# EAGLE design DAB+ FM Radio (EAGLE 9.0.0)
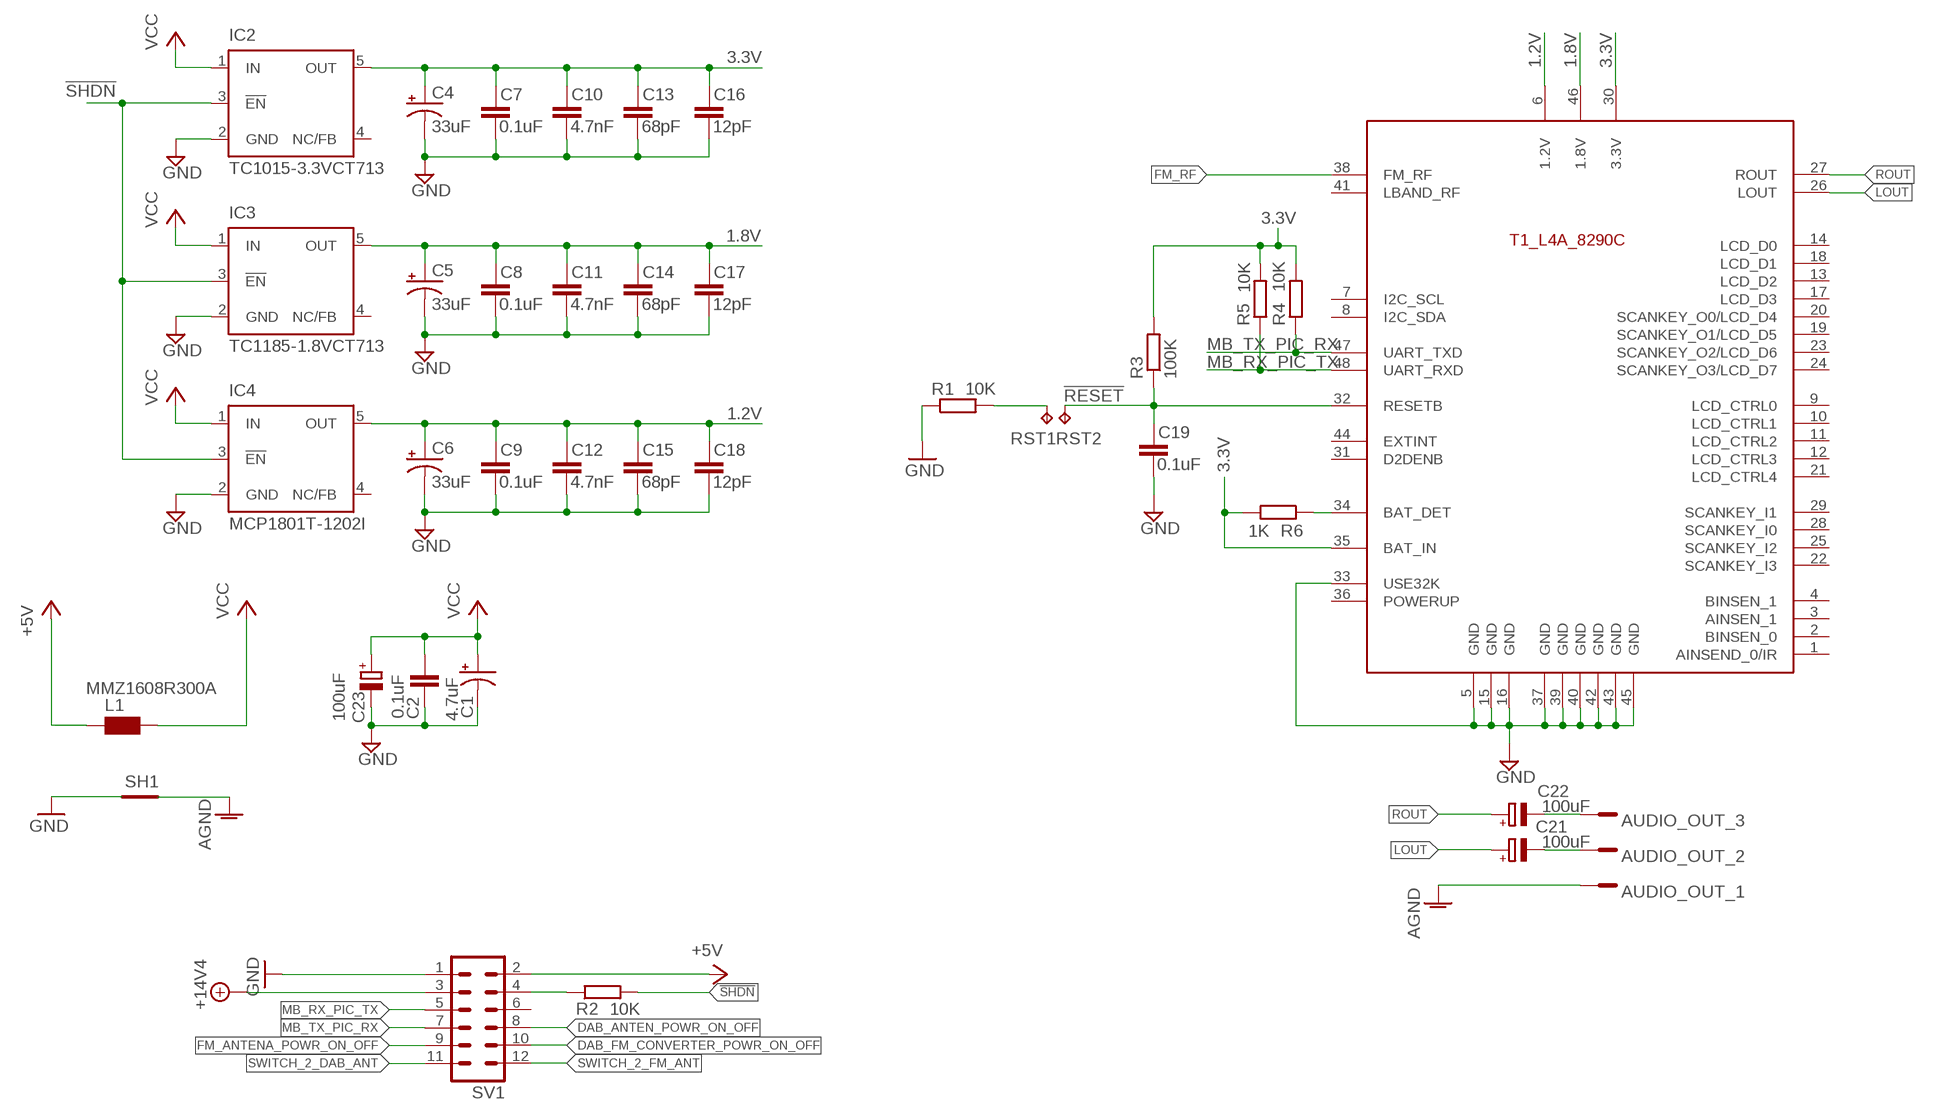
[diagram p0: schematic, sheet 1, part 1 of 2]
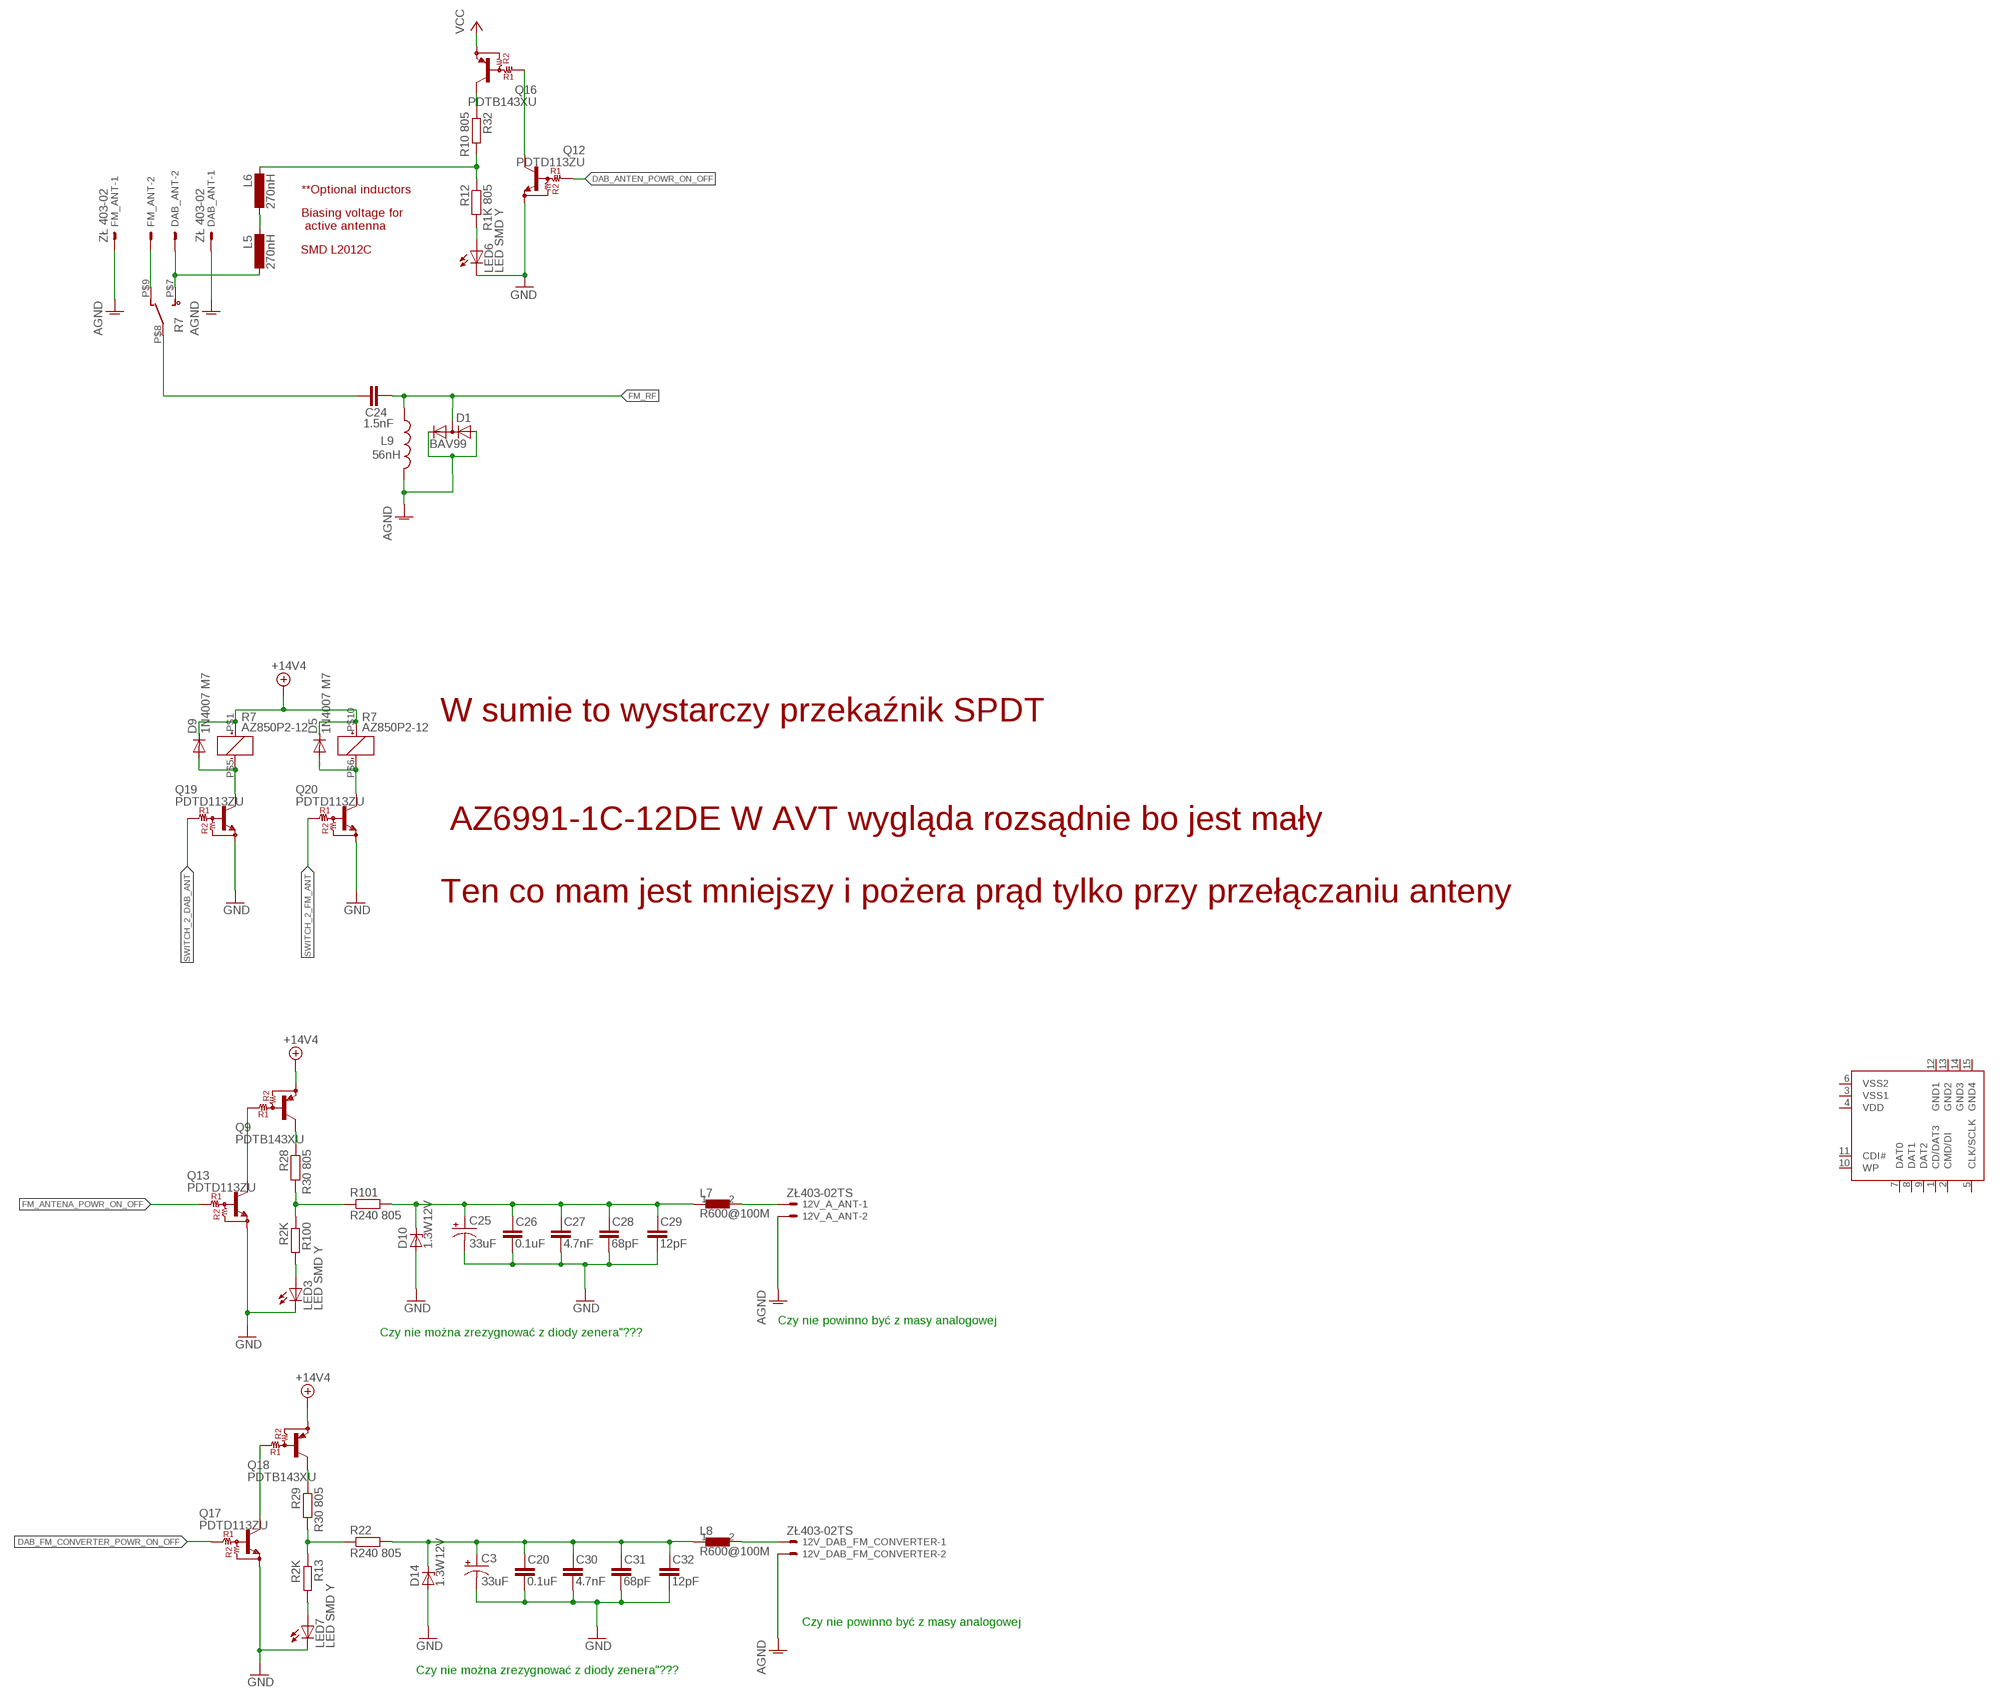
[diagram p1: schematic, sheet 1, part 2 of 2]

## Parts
12V_A_ANT  ZŁ403-02TS  22-23-2021  [22-23-2021]
12V_DAB_FM_CONVERTER  ZŁ403-02TS  22-23-2021  [22-23-2021]
AUDIO_OUT  JST_3_PIN_B3B-PH-KS  [B3B-PH-KS]
C1  4.7uF  CAP_POL1206  [EIA3216]
C2  0.1uF  C-EUC0603  [C0603]
C3  33uF  CAP_POL1206  [EIA3216]
C4  33uF  CAP_POL1206  [EIA3216]
C5  33uF  CAP_POL1206  [EIA3216]
C6  33uF  CAP_POL1206  [EIA3216]
C7  0.1uF  C-EUC0603  [C0603]
C8  0.1uF  C-EUC0603  [C0603]
C9  0.1uF  C-EUC0603  [C0603]
C10  4.7nF  C-EUC0603  [C0603]
C11  4.7nF  C-EUC0603  [C0603]
C12  4.7nF  C-EUC0603  [C0603]
C13  68pF  C-EUC0603  [C0603]
C14  68pF  C-EUC0603  [C0603]
C15  68pF  C-EUC0603  [C0603]
C16  12pF  C-EUC0603  [C0603]
C17  12pF  C-EUC0603  [C0603]
C18  12pF  C-EUC0603  [C0603]
C19  0.1uF  C-EUC0603  [C0603]
C20  0.1uF  C-EUC0603  [C0603]
C21  100uF  CPOL-EUD  [PANASONIC_D]
C22  100uF  CPOL-EUD  [PANASONIC_D]
C23  100uF  CPOL-EUD  [PANASONIC_D]
C24  1.5nF  C-EUC0603  [C0603]
C25  33uF  CAP_POL1206  [EIA3216]
C26  0.1uF  C-EUC0603  [C0603]
C27  4.7nF  C-EUC0603  [C0603]
C28  68pF  C-EUC0603  [C0603]
C29  12pF  C-EUC0603  [C0603]
C30  4.7nF  C-EUC0603  [C0603]
C31  68pF  C-EUC0603  [C0603]
C32  12pF  C-EUC0603  [C0603]
D1  BAV99  BAV199  [SOT23]
D5  1N4007 M7  CGRM4001-G  [SOD-123_MINI-SMA]
D9  1N4007 M7  CGRM4001-G  [SOD-123_MINI-SMA]
D10  1.3W12V  ZENER-DIODEZD-2.5  [ZDIO-2.5]
D14  1.3W12V  ZENER-DIODEZD-2.5  [ZDIO-2.5]
DAB_ANT  ZŁ 403-02  22-27-2021-02  [6410-02]
FM_ANT  ZŁ 403-02  22-27-2021-02  [6410-02]
IC2  TC1015-3.3VCT713  TPS77001  [SOT23-DBV]
IC3  TC1185-1.8VCT713  TPS77001  [SOT23-DBV]
IC4  MCP1801T-1202I  TPS77001  [SOT23-DBV]
L1  MMZ1608R300A  WE-CBF_0603  [0603]
L5  270nH  L-EUL2012C  [L2012C]
L6  270nH  L-EUL2012C  [L2012C]
L7  R600@100M  FERRITR0805  [R0805]
L8  R600@100M  FERRITR0805  [R0805]
L9  56nH  INDUCTOR0603  [0603]
LED3  LED SMD Y  LED  [SMARTLED-TTW]
LED6  LED SMD Y  LED  [SMARTLED-TTW]
LED7  LED SMD Y  LED  [SMARTLED-TTW]
Q9  PDTB143XU  [SOT-23]
Q12  PDTD113ZU  [SOT-23]
Q13  PDTD113ZU  [SOT-23]
Q16  PDTB143XU  [SOT-23]
Q17  PDTD113ZU  [SOT-23]
Q18  PDTB143XU  [SOT-23]
Q19  PDTD113ZU  [SOT-23]
Q20  PDTD113ZU  [SOT-23]
R1  10K  R-EU_R0603  [R0603]
R2  10K  R-EU_R0603  [R0603]
R3  100K  R-EU_R0603  [R0603]
R4  10K  R-EU_R0603  [R0603]
R5  10K  R-EU_R0603  [R0603]
R6  1K  R-EU_R0603  [R0603]
R7  AZ850P2-12  [AZ850-2C]
R12  R1K 805  R-EU_R0805  [R0805]
R13  R2K  R-EU_R0805  [R0805]
R22  R240 805  R-EU_M0805  [M0805]
R28  R30 805  R-EU_R0805  [R0805]
R29  R30 805  R-EU_R0805  [R0805]
R32  R10 805  R-EU_R0805  [R0805]
R100  R2K  R-EU_R0805  [R0805]
R101  R240 805  R-EU_M0805  [M0805]
RST1  TPB1,27  [B1,27]
RST2  TPB1,27  [B1,27]
SH1  SHORT-HT5  [SHORT_TOP-50]
SV1  MA06-2  [MA06-2]
U$1  T1_L4A_8290C/T2_L4A_8650C  T1_L4A_8290C  [T1_L4A]
U$6  ZŁ KART SD  SDCARDVAR2  [SDCMF-10915W010]

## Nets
1.2V: C6.A(+) C9.1 C12.1 C15.1 C18.1 IC4.5(OUT) U$1.6(1.2V)
1.8V: C5.A(+) C8.1 C11.1 C14.1 C17.1 IC3.5(OUT) U$1.46(1.8V)
3.3V: C4.A(+) C7.1 C10.1 C13.1 C16.1 IC2.5(OUT) R3.2 R4.2 R5.2 R6.2 U$1.30(3.3V) U$1.35(BAT_IN)
!RESET!: C19.1 R3.1 RST2.TP U$1.32(RESETB)
!SHDN!: IC2.3(!EN) IC3.3(!EN) IC4.3(!EN) R2.2
+5V: L1.1 SV1.2
+12V: D5.C D9.C Q9.2(E) Q18.2(E) R7.P$1(S$1:+) R7.P$10(R$2:+) SV1.3 ; supply symbol labelled +14V4
AGND: 12V_A_ANT.2 12V_DAB_FM_CONVERTER.2 AUDIO_OUT.P$1 D1.1(A) D1.2(C) DAB_ANT.1 FM_ANT.1 L9.2 SH1.2
DAB_ANTEN_POWR_ON_OFF: Q12.1(B) SV1.8
DAB_FM_CONVERTER_POWR_ON_OFF: Q17.1(B) SV1.10
FM_ANTENA_POWR_ON_OFF: Q13.1(B) SV1.9
FM_RF: C24.2 D1.3(AC) L9.1 U$1.38(FM_RF)
GND: C1.C(-) C2.2 C3.C(-) C4.C(-) C5.C(-) C6.C(-) C7.2 C8.2 C9.2 C10.2 C11.2 C12.2 C13.2 C14.2 C15.2 C16.2 C17.2 C18.2 C19.2 C20.2 C23.- C25.C(-) C26.2 C27.2 C28.2 C29.2 C30.2 C31.2 C32.2 D10.A D14.A IC2.2(GND) IC3.2(GND) IC4.2(GND) LED3.C@1(C) LED6.C@1(C) LED7.C@1(C) Q12.2(E) Q13.2(E) Q17.2(E) Q19.2(E) Q20.2(E) R1.1 SH1.1 SV1.1 U$1.5(GND) U$1.15(GND) U$1.16(GND) U$1.33(USE32K) U$1.37(GND) U$1.39(GND) U$1.40(GND) U$1.42(GND) U$1.43(GND) U$1.45(GND)
LOUT: C21.+ U$1.26(LOUT)
MB_RX_PIC_TX: R5.1 SV1.5 U$1.48(UART_RXD)
MB_TX_PIC_RX: R4.1 SV1.7 U$1.47(UART_TXD)
N$1: D5.A Q20.3(C) R7.P$6(R$2:-)
N$2: D9.A Q19.3(C) R7.P$5(S$1:-)
N$3: R6.1 U$1.34(BAT_DET)
N$4: C24.1 R7.P$8
N$5: DAB_ANT.2 L5.2 R7.P$7
N$6: AUDIO_OUT.P$3 C22.-
N$7: FM_ANT.2 R7.P$9
N$8: AUDIO_OUT.P$2 C21.-
N$9: L6.1 R12.1 R32.2
N$10: R2.1 SV1.4
N$12: L5.1 L6.2
N$13: R1.2 RST1.TP
N$20: Q12.3(C) Q16.1(B)
N$23: LED6.A@1(A) R12.2
N$25: Q17.3(C) Q18.1(B)
N$26: R13.1 R22.1 R29.2
N$27: LED7.A@1(A) R13.2
N$29: C3.A(+) C20.1 C30.1 C31.1 C32.1 D14.C L8.1 R22.2
N$30: 12V_DAB_FM_CONVERTER.1 L8.2
N$33: Q16.3(C) R32.1
N$34: Q9.3(C) R28.1
N$35: Q18.3(C) R29.1
N$85: Q9.1(B) Q13.3(C)
N$87: R28.2 R100.1 R101.1
N$88: LED3.A@1(A) R100.2
N$91: C25.A(+) C26.1 C27.1 C28.1 C29.1 D10.C L7.1 R101.2
N$92: 12V_A_ANT.1 L7.2
ROUT: C22.+ U$1.27(ROUT)
SWITCH_2_DAB_ANT: Q19.1(B) SV1.11
SWITCH_2_FM_ANT: Q20.1(B) SV1.12
VCC: C1.A(+) C2.1 C23.+ IC2.1(IN) IC3.1(IN) IC4.1(IN) L1.2 Q16.2(E)
Unconnected: IC2.4(NC/FB) IC3.4(NC/FB) IC4.4(NC/FB) R7.P$2 R7.P$3 R7.P$4 SV1.6 U$1.1(AINSEND_0/IR) U$1.2(BINSEN_0) U$1.3(AINSEN_1) U$1.4(BINSEN_1) U$1.7(I2C_SCL) U$1.8(I2C_SDA) U$1.9(LCD_CTRL0) U$1.10(LCD_CTRL1) U$1.11(LCD_CTRL2) U$1.12(LCD_CTRL3) U$1.13(LCD_D2) U$1.14(LCD_D0) U$1.17(LCD_D3) U$1.18(LCD_D1) U$1.19(SCANKEY_O1/LCD_D5) U$1.20(SCANKEY_O0/LCD_D4) U$1.21(LCD_CTRL4) U$1.22(SCANKEY_I3) U$1.23(SCANKEY_O2/LCD_D6) U$1.24(SCANKEY_O3/LCD_D7) U$1.25(SCANKEY_I2) U$1.28(SCANKEY_I0) U$1.29(SCANKEY_I1) U$1.31(D2DENB) U$1.36(POWERUP) U$1.41(LBAND_RF) U$1.44(EXTINT) U$6.1(CD/DAT3) U$6.2(CMD/DI) U$6.5(CLK/SCLK) U$6.7(DAT0) U$6.8(DAT1) U$6.9(DAT2) U$6.10(WP) U$6.11(CDI#)

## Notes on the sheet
- **Optional inductors
- Biasing voltage for
   active antenna
- SMD L2012C
- W sumie to wystarczy przekaźnik SPDT
  
  
   AZ6991-1C-12DE W AVT wygląda rozsądnie bo jest mały
  
  Ten co mam jest mniejszy i pożera prąd tylko przy przełączaniu anteny
- Czy nie powinno być z masy analogowej
- Czy nie można zrezygnować z diody zenera"???
- Czy nie powinno być z masy analogowej
- Czy nie można zrezygnować z diody zenera"???

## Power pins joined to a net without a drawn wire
GND1: U$6.12(GND1)
GND2: U$6.13(GND2)
GND3: U$6.14(GND3)
GND4: U$6.15(GND4)
VDD: U$6.4(VDD)
VSS1: U$6.3(VSS1)
VSS2: U$6.6(VSS2)

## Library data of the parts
12V_A_ANT 12V_DAB_FM_CONVERTER = con-molex:22-23-2021: .100" (2.54mm) Center Header - 2 Pin; MF: MOLEX; MPN: 22-23-2021; OC_FARNELL: 1462926; OC_NEWARK: 25C3832
AUDIO_OUT = conn-JST:JST_3_PIN_
C1 C3-C6 C25 = SparkFun:CAP_POL: Capacitor Polarized
C2 C7-C20 C24 C26-C32 = rcl:C-EU: CAPACITOR, European symbol
C21-C23 = rcl:CPOL-EU: POLARIZED CAPACITOR, European symbol
D1 = diode:BAV199: DIODE low-leakage double diode
D5 D9 = diode:CGRM400*-G: Molded plasitc,JEDEC SOD-123/Mini SMA
D10 D14 = diode:ZENER-DIODE: Z-Diode
DAB_ANT FM_ANT = con-molex:22-?-02: CONNECTOR; OC_FARNELL: unknown; OC_NEWARK: unknown
IC2-IC4 = texas:TPS770*: ULTRALOW-POWER 50-mA LOW-DROPOUT LINEAR REGULATORS 50-mA Low-Dropout Regulator Source: http://focus.ti.com/lit/ds/symlink/tps77001.pdf; MF: TEXAS INSTRUMENTS; MPN: TPS77001DBVT; OC_FARNELL: 8461554; OC_NEWARK: 77C1171
L1 = wuerth-elektronik:WE-CBF: SMD EMI Suppression Ferrite Beads
L5 L6 = resistor:L-EU: INDUCTOR, European symbol
L7 L8 = ferrit_bear:FERRIT
L9 = SparkFun:INDUCTOR: Inductors
LED3 LED6 LED7 = adafruit:LED: LED
Q9 Q16 Q18 = pre-bias-transistor:PDTB: PNP Resistor-Equipped Transistor (RET) family in a very small SOT323 (SC-70) Surface-Mounted Device (SMD) plastic package. VCC = -50 IC (max) = -500mA; R1: 4.7 kOhm; R2: 10 kOhm
Q12 Q13 Q17 Q19 Q20 = pre-bias-transistor:PDTD: Pre biase NPN transistor NPN Resistor-Equipped Transistor (RET) family in a very small SOT323 (SC-70) Surface-Mounted Device (SMD) plastic package. VCC = 50V Ic (max) = 500 mA; R1: 1 kOhm; R2: 10 kOhm
R1-R6 R12 R13 R22 R28 R29 R32 R100 R101 = rcl:R-EU_: RESISTOR, European symbol
R7 = relay_silelis:AZ850P2-12
RST1 RST2 = testpad:TP: Test pad
SH1 = shorts-old:SHORT-H: Short between two nets; BOM: no
SV1 = con-lstb:MA06-2: PIN HEADER; OC_FARNELL: unknown; OC_NEWARK: unknown
U$1 = Monkey:T1_L4A_8290C
U$6 = kingfont_sdcmf10915w010_covek:SDCARD: SD card connector KINGFONT SDCMF-10915W010

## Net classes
0 default: clearance 0.203 mm

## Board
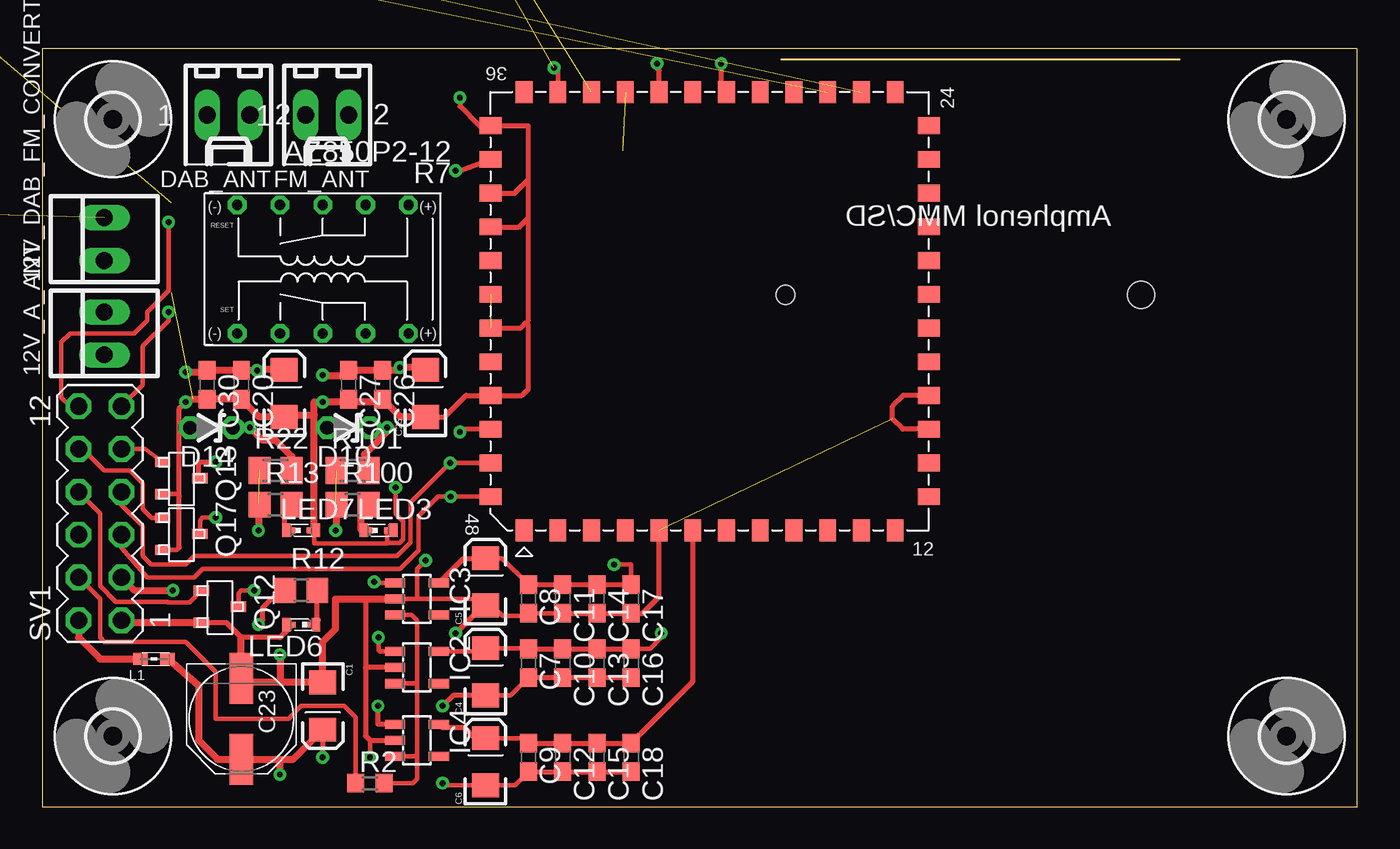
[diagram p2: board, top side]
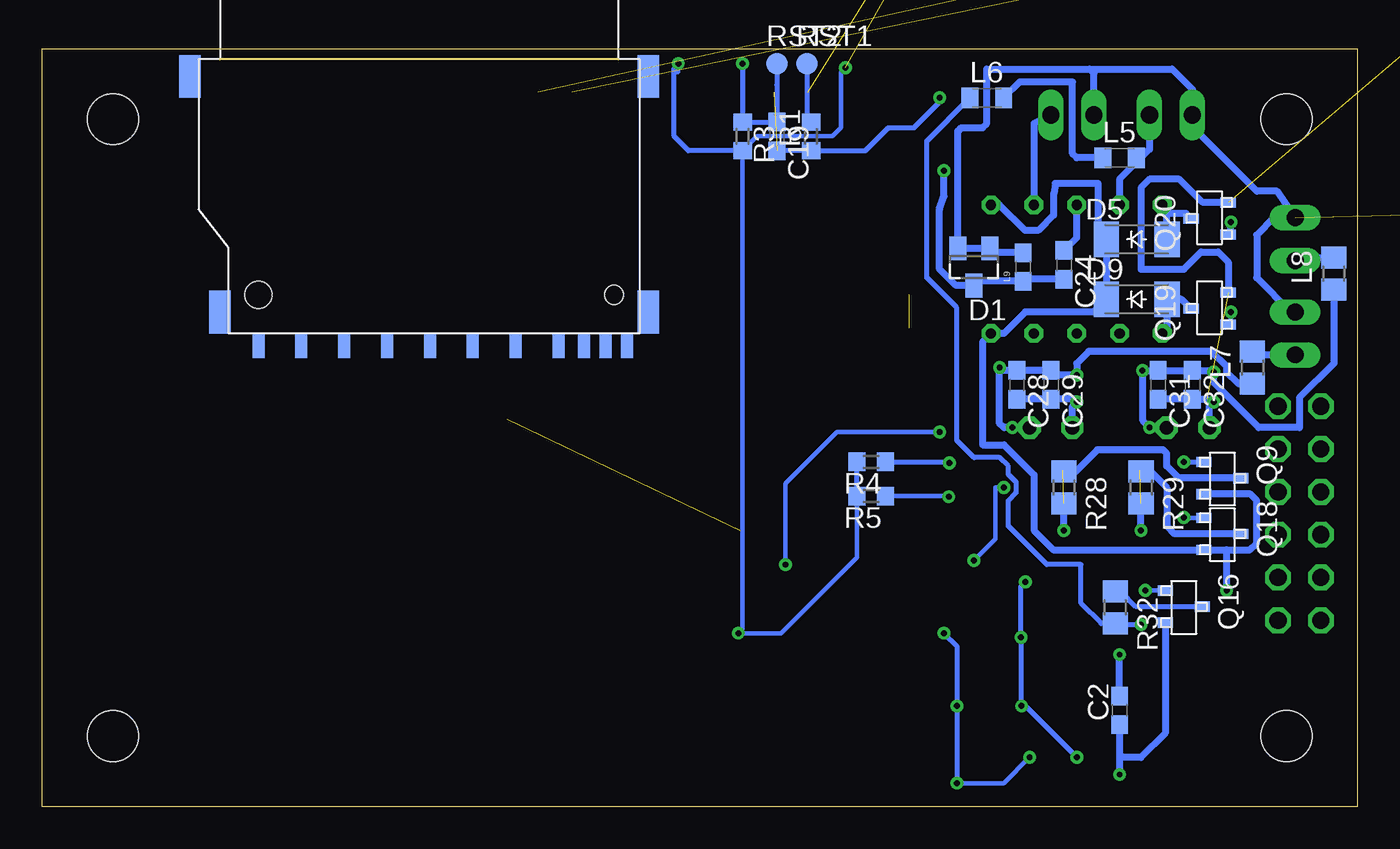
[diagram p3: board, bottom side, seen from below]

Size 77.98 x 44.96 mm. Coordinates in mm from the lower left corner, seen from the top.
Outline: 0,0 77.98,0 77.98,44.96 0,44.96 0,0
Copper layers (1*16): Top 0.035mm / dielectric 1.5mm / Bottom 0.035mm
Design rules "default": minimum track width 6mil, minimum drill 0.35mm, track to track 6mil, track to pad 6mil, pad to pad 6mil, via to via 6mil, smd to smd 6mil, copper to edge 40mil, drill to drill 6mil, minimum pad ring 10mil, minimum via ring 8mil, stop-mask expansion 4mil, vias tented up to drill 0mil, thermal gap 10mil

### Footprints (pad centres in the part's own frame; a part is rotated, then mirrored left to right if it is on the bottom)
22-23-2021 = drill 1 long: 1 -1.27,0; 2 1.27,0
B3B-PH-KS = drill 0.75 pad 1.2 square: P$1 -2,1.7; P$2 -4,1.7; P$3 -6,1.7
EIA3216 = smd 1.4 x 1.6: A 1.4,0; C -1.4,0
C0603 = smd 1.1 x 1: 1 -0.85,0; 2 0.85,0
PANASONIC_D = smd 3 x 1.4: + 2.4,0; - -2.4,0
SOT23 = smd 1 x 1.4: 1 -0.95,-1.1; 2 0.95,-1.1; 3 0,1.1
SOD-123_MINI-SMA = smd 1.5 x 2.1: A 1.8,0; C -1.8,0
ZDIO-2.5 = drill 0.813 octagon: A 1.27,0; C -1.27,0
6410-02 = drill 1.016 long: 1 1.27,0; 2 -1.27,0
SOT23-DBV = smd 0.55 x 1.2: 1 -0.95,-1.3; 2 0,-1.3; 3 0.95,-1.3; 4 0.95,1.3; 5 -0.95,1.3
0603 = smd 0.85 x 0.7: 1 -0.9,0; 2 0.7,0
L2012C = smd 1 x 1.2: 1 -1,0; 2 1,0
R0805 = smd 1.3 x 1.5: 1 -0.95,0; 2 0.95,0
0603' = smd 1.1 x 1: 1 -0.85,0; 2 0.85,0
SMARTLED-TTW = smd 0.8 x 0.5: A 0,-0.875; C 0,0.875 | smd 0.35 x 0.35: A@1 0,-0.5; C@1 0,0.5
SOT-23 = smd 0.6 x 0.9: 1 -1,-1.1; 2 0.9,-1.1; 3 -0.05,1.1
R0603 = smd 1 x 1.1: 1 -0.85,0; 2 0.85,0
AZ850-2C = drill 0.6 octagon: P$1 -5.08,3.81; P$2 -2.54,3.81; P$3 0,3.81; P$4 2.54,3.81; P$5 5.08,3.81; P$6 5.08,-3.81; P$7 2.54,-3.81; P$8 0,-3.81; P$9 -2.54,-3.81; P$10 -5.08,-3.81
M0805 = smd 1.3 x 1.6: 1 -0.95,0; 2 0.95,0
B1,27 = smd 1.27 x 1.27: TP 0,0
SHORT_TOP-50 = smd 1.27 x 1.27: 1 0.635,0; 2 -0.635,0
MA06-2 = drill 1.016 octagon: 1 -6.35,-1.27; 2 -6.35,1.27; 3 -3.81,-1.27; 4 -3.81,1.27; 5 -1.27,-1.27; 6 -1.27,1.27; 7 1.27,-1.27; 8 1.27,1.27; 9 3.81,-1.27; 10 3.81,1.27; 11 6.35,-1.27; 12 6.35,1.27
T1_L4A = smd 1.3 x 1: 1 0,0; 2 0,-2; 3 0,-4; 4 0,-6; 5 0,-8; 6 0,-10; 7 0,-12; 8 0,-14; 9 0,-16; 10 0,-18; 11 0,-20; 12 0,-22; 25 26,-22; 26 26,-20; 27 26,-18; 28 26,-16; 29 26,-14; 30 26,-12; 31 26,-10; 32 26,-8; 33 26,-6; 34 26,-4; 35 26,-2; 36 26,0 | smd 1 x 1.3: 13 2,-24; 14 4,-24; 15 6,-24; 16 8,-24; 17 10,-24; 18 12,-24; 19 14,-24; 20 16,-24; 21 18,-24; 22 20,-24; 23 22,-24; 24 24,-24; 37 24,2; 38 22,2; 39 20,2; 40 18,2; 41 16,2; 42 14,2; 43 12,2; 44 10,2; 45 8,2; 46 6,2; 47 4,2; 48 2,2
3,0 = hole 3: 0,0
SDCMF-10915W010 = smd 0.711 x 1.422: 1 7.366,13.462; 2 4.826,13.462; 3 2.286,13.462; 4 -0.254,13.462; 5 -2.794,13.462; 6 -5.334,13.462; 7 -7.874,13.462; 8 -9.398,13.462; 9 9.906,13.462; 10 -11.938,13.462; 11 -10.668,13.462 | smd 1.27 x 2.54: 12 12.192,11.43; 13 13.97,-2.54; 14 -13.208,-2.54; 15 -13.208,11.43 | hole 1.6: 9.906,10.414 | hole 1.1: -11.176,10.414

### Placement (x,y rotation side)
12V_A_ANT  3.68,28.07 90 top
12V_DAB_FM_CONVERTER  3.68,33.66 90 top
AUDIO_OUT  not placed on the board
C1  16.64,5.97 270 top
C2  14.1,5.71 90 bottom
C3  14.35,24.51 90 top
C4  26.29,8 90 top
C5  26.29,13.34 90 top
C6  26.29,2.67 90 top
C7  28.83,8.51 270 top
C8  28.83,12.32 270 top
C9  28.83,2.92 270 top
C10  30.86,8.51 270 top
C11  30.86,12.32 270 top
C12  30.86,2.92 270 top
C13  32.89,8.51 270 top
C14  32.89,12.32 270 top
C15  32.89,2.92 270 top
C16  34.92,8.51 270 top
C17  34.92,12.32 270 top
C18  34.92,2.92 270 top
C19  34.42,39.75 270 bottom
C20  11.81,25.02 270 top
C21  not placed on the board
C22  not placed on the board
C23  11.81,5.21 270 top
C24  17.4,32.13 270 bottom
C25  22.73,24.51 90 top
C26  20.19,25.02 270 top
C27  18.16,25.02 270 top
C28  20.19,25.02 270 bottom
C29  18.16,25.02 270 bottom
C30  9.78,25.02 270 top
C31  11.81,25.02 270 bottom
C32  9.78,25.02 270 bottom
D1  22.73,32 180 bottom
D5  13.08,33.66 0 bottom
D9  13.08,30.1 0 bottom
D10  18.16,22.48 180 top
D14  10.03,22.48 180 top
DAB_ANT  11.05,41.02 180 top
FM_ANT  16.89,41.02 180 top
IC2  22.22,8.25 270 top
IC3  22.22,12.32 270 top
IC4  22.22,3.94 270 top
L1  6.73,8.76 0 top
L5  14.1,38.48 0 bottom
L6  21.97,42.04 0 bottom
L7  6.22,26.04 90 bottom
L8  1.4,31.62 90 bottom
L9  56nH  [0603']  19.81,32 90 bottom
LED3  19.94,16.38 270 top
LED6  15.37,10.79 90 top
LED7  15.37,16.38 270 top
Q9  8,19.43 270 bottom
Q12  10.54,11.81 270 top
Q13  8.25,19.43 270 top
Q16  10.29,11.81 270 bottom
Q17  8.25,16.13 270 top
Q18  8,16.13 270 bottom
Q19  8.76,29.59 90 bottom
Q20  8.76,34.92 90 bottom
R1  32.38,39.75 90 bottom
R2  19.43,1.4 0 top
R3  36.45,39.75 270 bottom
R4  28.83,20.45 180 bottom
R5  28.83,18.41 180 bottom
R6  not placed on the board
R7  16.64,31.88 180 top
R12  15.37,12.83 0 top
R13  13.84,17.91 0 top
R22  13.84,19.94 0 top
R28  17.4,18.92 270 bottom
R29  12.83,18.92 270 bottom
R32  14.35,11.81 270 bottom
R100  18.41,17.91 0 top
R101  18.41,19.94 0 top
RST1  32.64,44.07 0 bottom
RST2  34.42,44.07 0 bottom
SH1  not placed on the board
SV1  3.43,17.4 90 top
U$1  28.57,16.38 90 top
U$2  [3,0]  4.19,40.77 0 top
U$3  [3,0]  4.19,4.19 0 top
U$4  [3,0]  73.79,40.77 0 top
U$5  [3,0]  73.79,4.19 0 top
U$6  55.24,40.77 180 bottom

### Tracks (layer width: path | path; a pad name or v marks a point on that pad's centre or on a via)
1.2V
  Top 0.254: C6.A 28.53,4.07 C9.1
  Top 0.305: IC4.5 23.71,4.7 25.02,4.7 25.65,4.07 C6.A 26.58,3.77 | C9.1 C12.1 C15.1 C18.1 38.57,7.42 U$1.6
1.8V  (via drill 0.35)
  Top 0.254: C5.A 27.26,14.73 C8.1 | C17.1 34.92,14.35 v33.91,14.35 | v24.77,22.22 24.92,22.38 U$1.46
  Top 0.305: 26.16,14.61 C5.A | C5.A 26.41,14.73 | C8.1 C11.1 C14.1 C17.1 | IC3.5 24.99,14.73 C5.A
  Bottom 0.254: v33.91,14.35 33.91,19.18 30.86,22.22 v24.77,22.22
3.3V  (via drill 0.35)  (1 unrouted)
  Top 0.254: IC2.5 26.09,9.21 C4.A 28.79,9.4 | U$1.35 30.57,43.59 v30.35,43.81 v30.35,43.82 | C16.1 36.03,9.36 36.7,10.03 v36.7,10.29
  Top 0.305: 28.79,9.4 C7.1 C10.1 C13.1 C16.1 | v40.26,44.07 40.26,42.7 U$1.30
  Bottom 0.254: v30.35,43.82 30.61,43.56 30.61,40.26 31.11,39.75 35.6,39.75 R3.2 36.45,10.54 v36.7,10.29 34.16,10.29 29.68,14.77 R5.2
  Bottom 0.305: R5.2 R4.2 | R3.2 39.66,38.9 40.51,39.75 40.51,43.79 40.29,43.56 v40.26,44.07
!RESET!  (via drill 0.35)
  Top 0.305: U$1.32 36.57,43.66 36.45,43.79 v36.45,44.07
  Bottom 0.305: v36.45,44.07 R3.1 C19.1 34.42,42.8 RST2.TP
!SHDN!
  Top 0.254: R2.2 21.97,1.4 22.22,1.65 22.22,3.17 | 22.22,3.17 22.22,7.24 | 22.22,7.24 22.22,11.05 21.9,11.37 IC3.3 | IC2.3 22.16,7.3 22.22,7.24 | IC4.3 22.16,2.99 22.22,3.17
+5V
  Top 0.406: SV1.2 2.16,10.03 3.43,8.76 L1.1
+12V  (via drill 0.35)
  Top 0.406: SV1.3 5.46,12.83 v7.75,12.83
  Bottom 0.406: D5.C D9.C 15.62,29.36 15.62,29.34 19.68,29.34 20.95,28.07 R7.P$1 22.22,27.56 22.22,21.46 20.95,21.46 19.18,19.68 19.18,16.38 18.02,15.23 Q18.2 7.75,15.23 | D5.C 14.88,34.44 | R7.P$10 21.21,35.69 19.68,34.16 18.92,34.16 18.01,35.08 18.01,36.34 18,36.36 17.91,36.96 15.37,36.96 15.37,34.67 14.88,34.19 D5.C | 7.75,15.23 6.36,15.23 5.97,15.62 5.97,18.16 6.34,18.53 Q9.2 | v7.75,12.83 7.75,15.23
AGND  (2 unrouted)
  Bottom 0.406: L9.2 21.53,32.85 D1.1 D1.2 | 23.75,33.1 D1.2 | 12V_A_ANT.2 3.94,29.34 5.97,31.37 5.97,33.91 4.95,34.92 12V_DAB_FM_CONVERTER.2 4.75,36.5 5.96,36.5 9.78,40.32 DAB_ANT.1 9.78,42.55 10.97,43.74 15.88,43.74 | 15.88,43.74 21.97,43.74 21.97,40.51 22.22,40.26 23.49,40.26 23.68,40.07 D1.2 | FM_ANT.1 15.62,43.48 15.88,43.74
DAB_ANTEN_POWR_ON_OFF
  Top 0.254: SV1.8 3.43,17.4 3.43,13.08 4.37,12.14 7.43,12.14 7.45,12.12 8.75,12.12 Q12.1
DAB_FM_CONVERTER_POWR_ON_OFF
  Top 0.254: SV1.10 2.41,21.21 3.68,19.94 5.21,19.94 5.97,19.18 5.97,17.65 6.49,17.13 Q17.1
FM_ANTENA_POWR_ON_OFF
  Top 0.254: SV1.9 6.12,21.21 Q13.1
FM_RF  (via drill 0.35)
  Top 0.305: U$1.38 24.61,37.62 v24.51,37.72
  Bottom 0.406: C24.2 19.68,31.28 L9.1 22.48,31.15 D1.3 23.79,30.9 24.77,31.88 24.77,35.43 24.51,36.2 v24.51,37.72
GND  (via drill 0.35)  (5 unrouted)
  Top 0.254: LED7.C@1 16.13,16.13 16.13,15.62 20.44,15.62 | LED3.C@1 20.44,15.62 | 20.44,15.62 20.45,15.62 20.48,15.65 21.2,15.65 21.39,15.85 21.39,16.92 20.95,17.36 v20.95,18.92 | Q13.2 8.01,18.53 8.13,18.41 | Q17.2 7.99,15.23 8.13,15.37 | v22.73,14.61 22.22,14.1 22.22,12.32 IC3.2 25.9,12.32 C5.C | 26.67,11.93 27.3,11.3 28.66,11.3 C8.2 C11.2 | C4.C 27.77,6.6 C7.2 | C9.2 28.02,1.27 C6.C 23.88,1.27 v23.75,1.4 v23.75,1.39 | v19.43,2.92 19.43,3.94
  Top 0.305: Q17.2 7.1,15.23 | 7.38,18.53 Q13.2 | 8.13,15.37 8.13,18.41 8.13,23.62 v8.51,24 | LED6.C@1 14.11,10.03 11.81,10.03 10.93,10.91 Q12.2 | 20.7,12.32 IC3.2 | 19.18,12.32 19.18,8.25 | 19.18,8.25 19.18,4.19 19.43,3.94 IC4.2 | IC2.2 19.18,8.25 | C9.2 C12.2 C15.2 C18.2 | C7.2 C10.2 C13.2 C16.2 | 26.67,11.93 C5.C 26.16,11.93 v24.51,10.29 | C11.2 C14.2 C17.2 35.6,11.47 36.57,12.45 U$1.5 | U$1.16 51.05,24.38 50.42,23.75 50.42,22.99 51.02,22.38 U$1.15 | U$1.39 28,36.38 28.83,37.21 | 28.83,37.21 28.83,40.38 U$1.37 25.91,40.38 24.77,41.53 v24.77,42.04 | U$1.40 28.29,34.38 28.83,34.92 | 28.83,34.92 28.83,37.21 | U$1.43 28.38,28.38 28.7,28.7 | 28.83,34.92 28.83,28.83 28.7,28.7 | 28.7,28.7 28.83,28.57 28.83,24.77 28.45,24.38 U$1.45 25.14,24.38 23.87,23.11 C25.C | C4.C 24.38,6.6 v23.75,5.97
  Top 0.406: C27.2 arc-90 18,24 | 18,24 v16.64,24 16.13,24 16.13,23.24 | 18,24 20.03,24 arc90 C28.2 21.25,23.11 C25.C | C3.C 12.87,23.11 C31.2 C30.2 8.93,24.17 v8.51,24 | C3.C 14.73,23.49 | 16.13,16.13 16.13,23.24 | C3.C 14.48,23.24 16.13,23.24 | Q12.2 4.84,10.91 SV1.1 | 11.81,10.03 C23.- 12.05,7.37 14.1,7.37 | 14.1,7.37 C1.C 16.64,9.78 17.4,10.54 17.4,12.32 19.18,12.32 20.7,12.32 | v14.1,9.02 14.1,7.37
  Bottom 0.254: v22.73,14.61 21.46,15.88 21.46,18.92 v20.95,18.92 | v23.75,1.39 20.96,1.39 v19.43,2.92
  Bottom 0.305: C19.2 R1.1 29.17,38.9 27.81,40.26 26.29,40.26 24.77,41.78 v24.77,42.04 | v23.75,1.39 v23.75,5.97 23.75,9.52 v24.51,10.29
  Bottom 0.406: Q20.2 9.16,35.82 10.54,37.21 12.32,37.21 12.83,36.7 12.83,31.88 10.29,31.88 9.27,32.89 8.25,32.89 7.66,32.3 Q19.2 | C28.2 C27.2 16.8,24.17 arc90 v16.64,24 16.89,23.75 D10.A | 9.69,24.26 C30.2 | C30.2 C31.2 | C30.2 8.93,24.17 v8.51,24 8.76,23.75 D14.A | C2.2 v14.1,9.02
LOUT  (1 unrouted)
MB_RX_PIC_TX  (via drill 0.35)
  Top 0.254: U$1.48 v24.22,18.38 23.46,18.38 22.31,17.23 22.31,15.2 21.21,14.1 9.52,14.1 9.02,13.59 6.22,13.59 4.7,15.37 SV1.5
  Bottom 0.254: R5.1 24.26,18.41 v24.22,18.38
MB_TX_PIC_RX  (via drill 0.35)
  Top 0.254: U$1.47 v24.19,20.38 21.85,18.04 21.85,15.66 21.05,14.86 9.02,14.86 8.51,14.35 6.48,14.35 5.97,14.86 5.97,16.64 4.7,17.91 SV1.7
  Bottom 0.305: v24.19,20.38 24.26,20.45 R4.1
N$1
  Bottom 0.406: D5.A 11.28,35.18 | 11.28,35.18 11.28,35.41 R7.P$6 | Q20.3 10.17,35.18 11.28,35.18
N$2
  Bottom 0.406: R7.P$5 11.28,28.34 D9.A 10.42,30.1 Q19.3
N$3  (1 unrouted)
N$4
  Bottom 0.406: C24.1 16.64,33.74 R7.P$8
N$5
  Bottom 0.406: R7.P$7 14.1,37.21 13.1,38.21 L5.2 12.83,38.48 12.32,38.99 DAB_ANT.2
N$6  (1 unrouted)
N$7
  Bottom 0.406: FM_ANT.2 19.18,40.51 R7.P$9
N$8  (1 unrouted)
N$9  (via drill 0.35)
  Top 0.305: v12.83,10.79 13.08,11.05 13.08,11.81 14.1,12.83 R12.1
  Bottom 0.305: v12.83,10.79 14.29,10.79 R32.2 15.18,10.86 16.38,12.07 16.38,14.35 18.41,14.35 20.7,16.64 20.7,18.14 20.22,18.62 20.22,19.23 20.7,19.71 20.7,20.19 21.21,20.7 22.73,20.7 23.75,21.72 23.75,29.59 25.53,31.37 25.53,39.48 L6.1
N$10
  Top 0.254: SV1.4 3.43,12.32 3.43,10.03 3.68,9.78 8.51,9.78 10.29,8 10.29,5.21 14.61,5.21 15.37,5.97 17.91,5.97 18.58,5.29 R2.1
N$12
  Bottom 0.406: L5.1 16.64,38.48 16.89,38.73 16.89,42.98 20.03,42.98 L6.2
N$13
  Bottom 0.305: RST1.TP 32.64,40.85 R1.2
N$20  (via drill 0.35)
  Top 0.254: Q12.3 11.64,12.66 11.81,12.83 v12.57,12.83
  Bottom 0.254: v12.57,12.83 12.56,12.81 Q16.1
N$23
  Top 0.305: LED6.A@1 16.13,10.79 16.38,11.05 16.32,11.11 R12.2
N$25  (via drill 0.35)
  Top 0.254: Q17.3 9.36,16.98 9.52,17.14 v10.29,17.14
  Bottom 0.254: Q18.1 10.27,17.13 v10.29,17.14
  Bottom 0.305: 9.12,17.14 Q18.1
N$26  (via drill 0.35)  (1 unrouted)
  Top 0.406: R13.1 12.83,17.84 v12.83,16.38
  Bottom 0.406: v12.83,16.38 R29.2
N$27
  Top 0.305: R13.2 arc90 14.35,17.46 14.35,16.38 LED7.A@1
N$29  (via drill 0.35)
  Top 0.406: v8.51,25.78 9.69,25.78 C32.1 C31.1 11.85,25.91 11.89,25.87 v12.74,25.87 12.78,25.91 C3.A | R22.2 14.79,20.77 13.84,21.72 13.08,21.72 v12.32,22.48
  Bottom 0.406: 1.22,30.49 L8.1 1.4,26.29 3.43,24.26 3.43,22.48 5.85,22.48 8.51,25.14 v8.51,25.78 8.6,25.87 C32.1 C31.1 v12.74,25.87 12.72,25.85 12.72,22.88 v12.32,22.48 D14.C
N$30
  Bottom 0.406: 12V_DAB_FM_CONVERTER.1 3.5,32.57 L8.2
N$33
  Bottom 0.305: Q16.3 13.13,11.86 14.03,12.76 R32.1
N$34
  Bottom 0.406: Q9.3 10.59,19.48 11.3,20.19 11.3,20.95 11.51,21.16 15.42,21.16 16.7,19.87 R28.1
N$35
  Bottom 0.406: Q18.3 10.84,16.18 11.3,16.64 11.3,18.92 12.25,19.87 R29.1 12.51,19.87
N$85  (via drill 0.35)
  Top 0.305: Q13.3 9.27,19.56 9.27,20.45 v10.29,20.45
  Bottom 0.305: v10.29,20.45 9.12,20.45 Q9.1
N$87  (via drill 0.35)  (1 unrouted)
  Top 0.406: R100.1 17.46,17.59 v17.4,16.38
  Bottom 0.406: v17.4,16.38 R28.2
N$88
  Top 0.406: R100.2 18.92,17.91 18.92,16.38 LED3.A@1
N$91  (via drill 0.35)
  Top 0.406: v16.64,25.59 16.64,25.53 17.82,25.53 arc90 C29.1 C28.1 21.04,25.87 v21.21,26.04 22.61,26.04 C25.A arc-90 22.69,25.87 | R101.2 19.11,20.89 20.7,22.48 v20.45,22.48
  Bottom 0.406: L7.1 7.05,25.08 7.72,25.76 7.72,26.11 8.67,27 15.93,27 16.64,26.29 v16.64,25.59 17.89,25.59 C29.1 C28.1 21.04,25.87 v21.21,26.04 21.21,22.73 20.95,22.48 v20.45,22.48 D10.C
N$92
  Bottom 0.406: 12V_A_ANT.1 6.04,26.8 L7.2
ROUT  (1 unrouted)
SWITCH_2_DAB_ANT  (via drill 0.35)
  Top 0.254: SV1.11 5.97,25.02 5.97,27.3 7.49,28.83 v7.49,29.34
  Bottom 0.254: v7.49,29.34 7.49,28.76 Q19.1
SWITCH_2_FM_ANT  (via drill 0.35)
  Top 0.254: v7.49,34.67 7.49,30.61 6.22,29.34 6.22,28.83 5.46,28.07 1.65,28.07 1.14,27.56 1.14,24.26 1.65,23.75 SV1.12
  Bottom 0.406: Q20.1 7.49,34.09 v7.49,34.67
VCC  (via drill 0.35)
  Top 0.254: IC3.1 19.75,13.27 v19.68,13.34 | IC2.1 20,9.21 19.94,9.27 v19.94,10.03
  Top 0.305: C1.A v16.64,2.92 | IC4.1 19.91,4.89 v19.91,5.97
  Top 0.406: L1.2 9.27,7.18 9.27,3.94 10.4,2.81 C23.+ 14.1,2.81 | 14.1,2.81 14.88,2.81 C1.A | v14.1,1.9 14.1,2.81
  Bottom 0.305: v19.68,13.34 19.94,13.08 v19.94,10.03 19.91,10 v19.91,5.97 19.68,5.97 v16.64,2.92
  Bottom 0.406: C2.1 14.1,2.92 | 14.1,2.92 v14.1,1.9 | Q16.2 11.39,4.36 12.83,2.92 14.1,2.92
